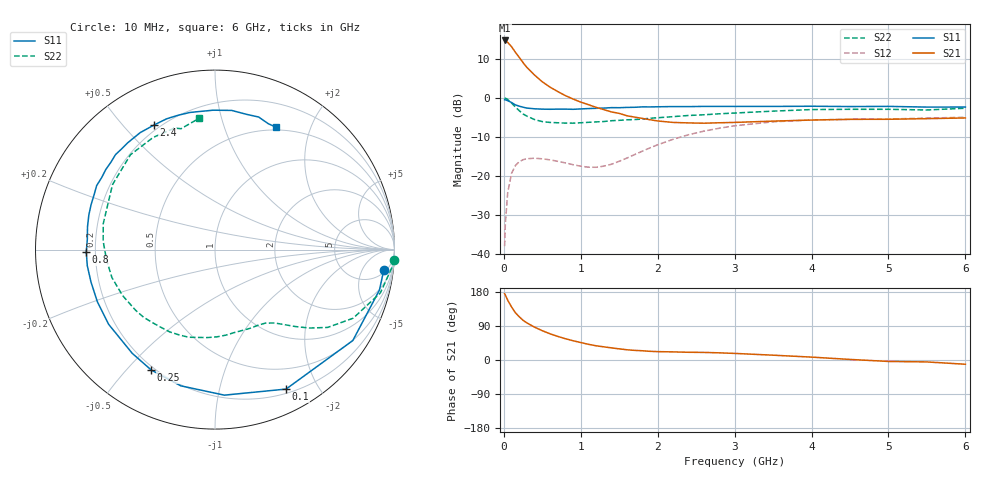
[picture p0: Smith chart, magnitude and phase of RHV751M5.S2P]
! SIEMENS Small Signal Semiconductors
! BFR106
! Si NPN RF Bipolar Junction Transistor in SOT23
! VCE = 0.75 V  IC = 1.5 mA
! Common Emitter S-Parameters:  August  1996
# GHz  S  MA  R  50
!  f  S11  S21  S12  S22
! GHz  MAG  ANG  MAG  ANG  MAG  ANG  MAG  ANG
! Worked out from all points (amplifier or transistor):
!   36 points, 10 MHz to 6 GHz, reference 50 ohm
!   highest |S21| = 14.7 dB at 10 MHz (marker M1)
!   |S21| within 3 dB of that: start of sweep to 149.3 MHz
!   unconditionally stable (mu >= 1): 788.8 MHz to end of sweep
!   at 250 MHz: K = 0.32, MSG = 12.4 dB, |S12| = -15.8 dB
!   at 1.4 GHz: K = 1.44, MAG = 2.7 dB, |S12| = -17.0 dB
!   at 6 GHz: K = 1.02, MAG = -1.0 dB, |S12| = -5.0 dB
!   S11 on the Smith chart (normalised r, x): 10 MHz: 6, -14; 100 MHz: 0.25, -1.60; 250 MHz: 0.19, -0.59; 800 MHz: 0.16, -0.01; 2.4 GHz: 0.18, +0.61; 6 GHz: 0.47, +1.52
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0.01  0.9474 -6.8  5.414 174.9  0.0127 87.5  0.9961 -3.2
0.02  0.9435 -13.8  5.38 171.2  0.0251 82.7  0.9895 -6.0
0.05  0.9199 -33.4  5.11 157.8  0.0611 70.6  0.9523 -14.7
0.1  0.8721 -63.0  4.516 140.1  0.108 55.0  0.8596 -26.4
0.15  0.8126 -86.3  3.824 124.7  0.1362 42.7  0.7633 -34.6
0.2  0.7826 -104.1  3.293 114.1  0.1526 34.5  0.6857 -39.6
0.25  0.7592 -117.9  2.82 104.7  0.1619 28.0  0.6222 -43.6
0.3  0.7393 -128.6  2.447 97.9  0.1666 23.6  0.5833 -46.2
0.4  0.7242 -144.9  1.95 86.6  0.1691 17.4  0.5269 -50.9
0.5  0.7169 -156.1  1.603 77.3  0.1661 13.4  0.4968 -55.5
0.6  0.7142 -165.4  1.371 69.2  0.1612 11.5  0.4847 -60.5
0.8  0.7172 -178.9  1.068 56.2  0.1473 11.9  0.4754 -71.3
1.1  0.7289 164.6  0.817 41.4  0.1298 22.8  0.4864 -89.0
1.6  0.7543 143.9  0.59 27.0  0.1697 49.4  0.5234 -118.8
2.2  0.7736 122.6  0.485 21.4  0.295 51.0  0.575 -153.5
2.4  0.7726 116.3  0.478 20.4  0.3375 47.6  0.595 -164.8
2.8  0.7763 105.3  0.48 18.9  0.4087 39.1  0.625 175.6
3.5  0.7768 90.8  0.504 12.7  0.4937 24.0  0.6762 147.6
4.5  0.7738 76.9  0.531 1.5  0.5314 6.3  0.7137 118.9
5  0.7777 71.8  0.532 -3.8  0.5364 -0.2  0.7135 108.4
5.5  0.7616 67.0  0.542 -5.1  0.5507 -3.3  0.6995 105.7
6  0.7624 63.3  0.553 -11.2  0.5646 -9.9  0.7364 97.0
